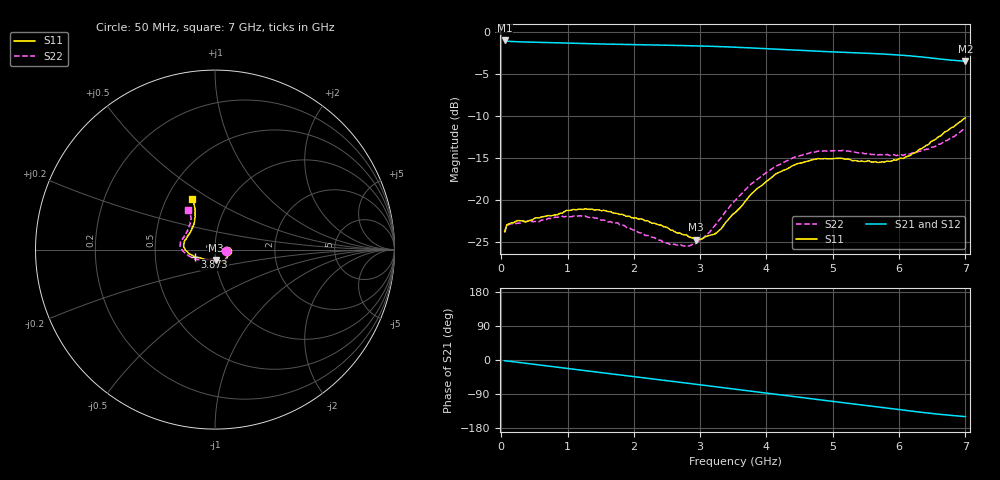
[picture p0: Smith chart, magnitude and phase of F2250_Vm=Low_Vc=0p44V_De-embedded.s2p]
! Integrated Device Technology
! Corporate Headquarters
! 6024 Silver Creek Valley Road
! San Jose, CA 95138  USA
! Phone:  1-408-284-8200
! Toll Free:  1-800-223-1366
! Webpage:  http://www.idt.com/
! Timing and RF Division
! 515 Groton Road, Suite 102
! Westford, MA 01886-6024
! Device:  F2250
! Description: Voltage Variable RF Attenuator
! Frequency:  50.0 -  6000.00 MHz
! Package:  3x3 mm Thin QFN Plastic Package: 16 pin
! Ports:  2 RF, 3 DC
!  Pin  1  = GND
!  Pin  2  = NC
!  Pin  3  = RF1  = Port 1
!  Pin  4  = NC
!  Pin  5  = GND
!  Pin  6  = GND
!  Pin  7  = GND
!  Pin  8  = GND
!  Pin  9  = NC
!  Pin 10  = RF2  = Port 2
!  Pin 11  = NC
!  Pin 12  = GND
!  Pin 13  = GND
!  Pin 14  = VCNTRL
!  Pin 15  = VDD
!  Pin 16  = VMODE
! Vcntrl:  0.440 Volts
! Vmode:  +0.000 Volts
! Vdd:  +3.30  Volts
! Current:  1.125 mA
! Data:  The device was measured on a the F2250 evaluation board which has
!  individual transmission lines to the RF pins.  Data was collected
!  using a calibrated network analyzer.  The evaluation board was
!  de-embedded using a TRL calibration technique.
!  The reference plane is the edge of the package pin.
! Misc:  SN 10
!  Action Tracker AT0258
! Date Measured:  2014-11-26
! Date:  2015-10-15  MJV
! Note:
!  Integrated Device Technology supplies this data as a sample of measured
!  data at the package pin for this product.  Your particular data for this
!  product may vary.
!  Data was taken at 25 degrees C.
!  Integrated Device Technology reserves the right to change this data at anytime.
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# GHz S dB R 50
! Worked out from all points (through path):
!   201 points, 50 MHz to 7 GHz, reference 50 ohm
!   highest |S21| = -1.02 dB at 50 MHz (marker M1); lowest = -3.5 dB at 7 GHz (marker M2)
!   group delay of S21, straight-line fit = 60.1 ps
!   lowest |S11| = -24.7 dB at 2.934 GHz (marker M3), VSWR 1.12, Z = 50.2 - j5.81 ohm
!   |S11| at or under -10 dB: start of sweep to end of sweep
!   |S22| runs from -25.5 to -11.5 dB; largest |S21 - S12| = 0.00041
!   S11 on the Smith chart (normalised r, x): 50 MHz: 1.14, -0.02; 3.873 GHz: 0.80, -0.07; 7 GHz: 0.67, +0.42
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0.05  -23.74 -8.5  -1.02 -1.8  -1.02 -1.8  -23.90 -9.1
0.08475  -22.95 -8.4  -1.10 -2.5  -1.09 -2.5  -23.05 -8.5
0.15425  -22.72 -10.5  -1.14 -4.0  -1.14 -4.0  -22.82 -10.2
0.6755  -21.92 -32.9  -1.27 -15.4  -1.27 -15.4  -22.35 -34.5
0.884  -21.59 -41.9  -1.31 -20.0  -1.31 -20.0  -21.96 -44.6
1.2315  -21.13 -51.8  -1.39 -27.4  -1.39 -27.4  -21.97 -57.3
1.75275  -21.61 -58.5  -1.48 -38.5  -1.48 -38.5  -22.71 -65.4
2.37825  -22.96 -59.8  -1.57 -51.8  -1.57 -51.8  -24.77 -69.6
2.552  -23.57 -63.6  -1.59 -55.6  -1.59 -55.7  -25.35 -75.4
2.83  -24.40 -76.9  -1.64 -61.7  -1.64 -61.7  -25.49 -93.1
2.93425  -24.74 -84.8  -1.66 -64.0  -1.66 -64.1  -25.19 -101.2
3.21225  -24.09 -113.1  -1.73 -70.2  -1.73 -70.2  -23.13 -125.5
3.525  -21.53 -141.4  -1.82 -77.2  -1.82 -77.2  -20.09 -144.4
3.8725  -18.56 -159.5  -1.95 -84.8  -1.95 -84.8  -17.48 -160.1
4.1505  -16.85 -170.0  -2.06 -90.9  -2.06 -90.9  -15.95 -170.1
4.4285  -15.81 -178.0  -2.17 -96.9  -2.17 -96.9  -14.90 -177.5
4.7065  -15.20 175.1  -2.27 -102.9  -2.27 -103.0  -14.34 176.4
5.15825  -15.08 164.3  -2.43 -112.7  -2.43 -112.7  -14.10 167.1
5.85325  -15.41 140.8  -2.68 -127.6  -2.68 -127.6  -14.70 151.7
6.166  -14.73 129.6  -2.85 -134.4  -2.85 -134.4  -14.54 142.8
6.444  -13.41 120.9  -3.06 -140.2  -3.06 -140.2  -13.95 133.4
7  -10.24 114.1  -3.50 -149.5  -3.50 -149.5  -11.46 123.9
